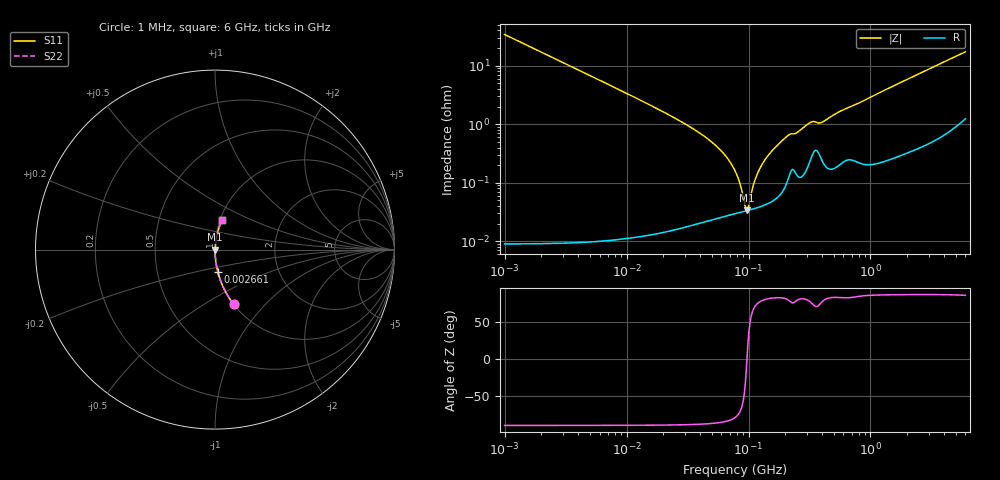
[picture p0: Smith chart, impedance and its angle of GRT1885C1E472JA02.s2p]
!Murata Part Number: GRT1885C1E472JA02
!These Parameters are Measured in Series Mode Connection
!Data Generated on Jun 19, 2026
!  o--ll--o
!Port1  Port2
!  o------o
!Operation Temp=25[degC], DC Bias Voltage=0[V]
!Freq. Start=1000[kHz] Stop=6[GHz] 401[Steps]
# Hz S RI R 50
!Freq.(Hz) S11(Real) S11(Imag) S21(Real) S21(Imag) S12(Real) S12(Imag) S22(Real) S22(Imag)
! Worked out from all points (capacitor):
!   401 points, 1 MHz to 6 GHz, reference 50 ohm
!   read as one part in series: C = 4.67 nF near 1.044 MHz
!   lowest |Z| = 33.8 mohm at 96.28 MHz (marker M1)
!   series resonance near 97.09 MHz, so ESL is about 580 pH
!   S11 on the Smith chart (normalised r, x): 1 MHz: 1.00, -0.68; 2.661 MHz: 1.00, -0.26; 6 GHz: 1.02, +0.34
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1000000  0.104 -0.3052  0.896 0.3052  0.896 0.3052  0.104 -0.3052
2660982  0.0162 -0.1258  0.9838 0.1258  0.9838 0.1258  0.0162 -0.1258
4293785  0.00632 -0.0787  0.9937 0.0787  0.9937 0.0787  0.00632 -0.0787
1.843659e7  0.000452 -0.0177  0.9995 0.0177  0.9995 0.0177  0.000452 -0.0177
3.316698e7  0.000265 -0.009  0.9997 0.009  0.9997 0.009  0.000265 -0.009
4.905945e7  0.000257 -0.00511  0.9997 0.00511  0.9997 0.00511  0.000257 -0.00511
6.368941e7  0.000276 -0.00301  0.9997 0.00301  0.9997 0.00301  0.000276 -0.00301
7.745967e7  0.000299 -0.00158  0.9997 0.00158  0.9997 0.00158  0.000299 -0.00158
8.450008e7  0.000311 -0.000965  0.9997 0.000965  0.9997 0.000965  0.000311 -0.000965
9.218041e7  0.000325 -0.000359  0.9997 0.000359  0.9997 0.000359  0.000325 -0.000359
9.627852e7  0.000333 -5.75e-05  0.9997 5.75e-05  0.9997 5.75e-05  0.000333 -5.75e-05
1.005588e8  0.000341 0.000245  0.9997 -0.000245  0.9997 -0.000245  0.000341 0.000245
1.096987e8  0.00036 0.000852  0.9996 -0.000852  0.9996 -0.000852  0.00036 0.000852
1.196694e8  0.000382 0.00147  0.9996 -0.00147  0.9996 -0.00147  0.000382 0.00147
1.455431e8  0.000454 0.00293  0.9995 -0.00293  0.9995 -0.00293  0.000454 0.00293
2.061188e8  0.00104 0.0061  0.999 -0.0061  0.999 -0.0061  0.00104 0.0061
2.506837e8  0.00137 0.0071  0.9986 -0.0071  0.9986 -0.0071  0.00137 0.0071
3.325952e8  0.00304 0.0106  0.997 -0.0106  0.997 -0.0106  0.00304 0.0106
4.045054e8  0.00241 0.0106  0.9976 -0.0106  0.9976 -0.0106  0.00241 0.0106
5.60538e8  0.0023 0.0163  0.9977 -0.0163  0.9977 -0.0163  0.0023 0.0163
1.428092e9  0.00418 0.0414  0.9958 -0.0414  0.9958 -0.0414  0.00418 0.0414
6e9  0.0398 0.1629  0.9602 -0.1629  0.9602 -0.1629  0.0398 0.1629
